(* Logix 5000 AddOnInstructionDefinition export Banner_TL70Pro_PD_v4; software revision 33.00 *)

TYPE Banner_TL70Pro_Adv_PD_Seg_v4 :   // Advanced process data set for a TL70 Pro Segment.
STRUCT
   Color_1 : SINT;   // 0 = Green, 1 = Red, 2 = Orange, 3 = Amber, 4 = Yellow, 5 = Lime Green, 6 = Spring Green, 7 = Cyan, 8 = Sky Blue, 9 = Blue, 10 = Violet, 11 = Magenta, 12 = Rose, 13 = White, 14 = Custom, 15 = Custom 2
   Color_1_Intensity : SINT;   // 0 = High, 1 = Low, 2 = Medium, 3 = Off, 4 = Custom
   Animation_Type : SINT;   // 0 = Off, 1 = Steady, 2 = Flash, 3 = Two Color, 4 = Half/Half, 5 = Half/Half Rotate, 6 = Chase, 7 = Intesnity Sweep
   Speed : SINT;   // 0 = Medium, 1 = Fast, 2 = Slow, 3 = Custom
   Pulse_Pattern : SINT;   // 0 = Normal, 1 = Strobe, 2 = Three Pulse, 3 = SOS, 4 = Random
   Color_2 : SINT;   // 0 = Green, 1 = Red, 2 = Orange, 3 = Amber, 4 = Yellow, 5 = Lime Green, 6 = Spring Green, 7 = Cyan, 8 = Sky Blue, 9 = Blue, 10 = Violet, 11 = Magenta, 12 = Rose, 13 = White, 14 = Custom, 15 = Custom 2
   Color_2_Instensity : SINT;   // 0 = High, 1 = Low, 2 = Medium, 3 = Off, 4 = Custom
END_STRUCT
END_TYPE

TYPE Banner_TL70Pro_Adv_PDIO_v4 :   // Advanced process data set for a TL70 Pro IO-Link unit.
STRUCT
   Segment_1 : Banner_TL70Pro_Adv_PD_Seg_v4;   // Advanced process data set for a TL70 Segment.
   Segment_2 : Banner_TL70Pro_Adv_PD_Seg_v4;   // Advanced process data set for a TL70 Segment.
   Segment_3 : Banner_TL70Pro_Adv_PD_Seg_v4;   // Advanced process data set for a TL70 Segment.
   Segment_4 : Banner_TL70Pro_Adv_PD_Seg_v4;   // Advanced process data set for a TL70 Segment.
   Segment_5 : Banner_TL70Pro_Adv_PD_Seg_v4;   // Advanced process data set for a TL70 Segment.
   Segment_6 : Banner_TL70Pro_Adv_PD_Seg_v4;   // Advanced process data set for a TL70 Segment.
   Audible : SINT;   // 0 = Off, 1 = On
END_STRUCT
END_TYPE

TYPE Banner_TL70Pro_Gauge_PD_v4 :   // Gauge mode process data set for a TL70 Pro IO-Link unit.
STRUCT
   Gauge_Value : INT;
   Audible : SINT;   // 0 = Off, 1 = On, 2 = Advanced
END_STRUCT
END_TYPE

TYPE Banner_TL70Pro_Level_PD_v4 :   // LeveL process data set for a TL70 Pro IO-Link unit.
STRUCT
   Level_Mode_Value : DINT;   // 0 to 65535. 0 = no lights on while 65535 = all lights on.
   Audible : SINT;   // 0 = Off, 1 = On
END_STRUCT
END_TYPE

TYPE Banner_TL70Pro_PDIO_v4 :   // Process data for a Banner TL70 Pro unit. This includes four process data types.
STRUCT
   Segment_PD : Banner_TL70Pro_Segment_PD_v4;
   Run_PD : Banner_TL70Pro_Run_PD_v4;
   Level_PD : Banner_TL70Pro_Level_PD_v4;
   Gauge_PD : Banner_TL70Pro_Gauge_PD_v4;
   Advanced_PD : Banner_TL70Pro_Adv_PDIO_v4;
   Transfer_Data : SINT[20];   // Data array to send the correct state of the process data output to the IO-Link master.
END_STRUCT
END_TYPE

TYPE Banner_TL70Pro_Run_PD_v4 :   // Run mode process data set for a TL70 Pro IO-Link unit.
STRUCT
   Animation : SINT;   // 0 = Off, 1 = Steady, 2 = Flash, 3 = Two Color, 4 = Half/Half, 5 = Half/Half Rotate, 6 = Chase, 7 = Intesnity Sweep, 8 = Scroll, 9 = Bounce, 10 = Demo
   Color_1 : SINT;   // 0 = Green, 1 = Red, 2 = Orange, 3 = Amber, 4 = Yellow, 5 = Lime Green, 6 = Spring Green, 7 = Cyan, 8 = Sky Blue, 9 = Blue, 10 = Violet, 11 = Magenta, 12 = Rose, 13 = White, 14 = Custom, 15 = Custom 2
   Color_1_Intensity : SINT;   // 0 = High, 1 = Low, 2 = Medium, 3 = Off, 4 = Custom
   Speed : SINT;   // 0 = Medium, 1 = Fast, 2 = Slow, 3 = Custom
   Pulse_Pattern : SINT;   // 0 = Normal, 1 = Strobe, 2 = Three Pulse, 3 = SOS, 4 = Random
   Color_2 : SINT;   // 0 = Green, 1 = Red, 2 = Orange, 3 = Amber, 4 = Yellow, 5 = Lime Green, 6 = Spring Green, 7 = Cyan, 8 = Sky Blue, 9 = Blue, 10 = Violet, 11 = Magenta, 12 = Rose, 13 = White, 14 = Custom, 15 = Custom 2
   Color_2_Intensity : SINT;   // 0 = High, 1 = Low, 2 = Medium, 3 = Off, 4 = Custom
   Scroll_Bounce_Style : SINT;   // 0 = Solid, 1 = Tail, 2 = Ripple
   Width_of_Color_1 : SINT;   // 1 to 100 percent
   Direction : SINT;   // 0 = Up, 1 = Down
   Audible : SINT;   // 0 = Off, 1 = On
END_STRUCT
END_TYPE

TYPE Banner_TL70Pro_Segment_PD_v4 :   // Basic process data set for a TL70 Pro IO-Link unit.
STRUCT
   Segment_1 : SINT;   // 0 = Off, 1 = On, 2 = Flash, 3 = Animation Type
   Segment_2 : SINT;   // 0 = Off, 1 = On, 2 = Flash, 3 = Animation Type
   Segment_3 : SINT;   // 0 = Off, 1 = On, 2 = Flash, 3 = Animation Type
   Segment_4 : SINT;   // 0 = Off, 1 = On, 2 = Flash, 3 = Animation Type
   Segment_5 : SINT;   // 0 = Off, 1 = On, 2 = Flash, 3 = Animation Type
   Segment_6 : SINT;   // 0 = Off, 1 = On, 2 = Flash, 3 = Animation Type
   Audible : SINT;   // 0 = Off, 1 = On
END_STRUCT
END_TYPE

ADD_ON_INSTRUCTION Banner_TL70Pro_Adv_PD_v4   (* revision 4.0, vendor Banner Engineering *)
// AOI converts the Advanced process and places it into the correct bytes for transfer to the IO-Link master.
VAR_IN_OUT
   Segment : Banner_TL70Pro_Adv_PD_Seg_v4; {required}
   Byte_1 : SINT; {required}
   Byte_2 : SINT; {required}
   Byte_3 : SINT; {required}
END_VAR

ROUTINE Logic   (* ladder *)
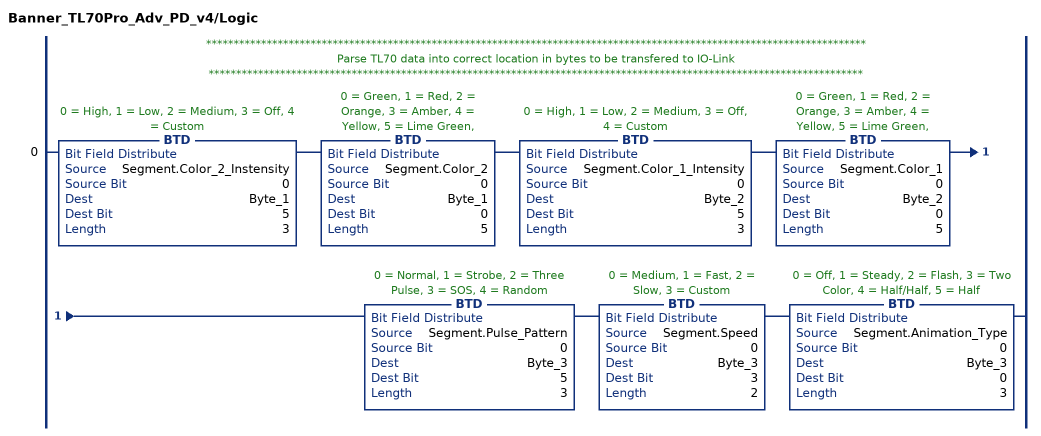
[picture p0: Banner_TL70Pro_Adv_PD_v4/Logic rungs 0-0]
   // ************************************************************************************************************************
   // Parse TL70 data into correct location in bytes to be transfered to IO-Link
   // ***********************************************************************************************************************
   0: BTD(Segment.Color_2_Instensity,0,Byte_1,5,3)BTD(Segment.Color_2,0,Byte_1,0,5)BTD(Segment.Color_1_Intensity,0,Byte_2,5,3)BTD(Segment.Color_1,0,Byte_2,0,5)BTD(Segment.Pulse_Pattern,0,Byte_3,5,3)BTD(Segment.Speed,0,Byte_3,3,2)BTD(Segment.Animation_Type,0,Byte_3,0,3);
END_ROUTINE
END_ADD_ON_INSTRUCTION

ADD_ON_INSTRUCTION Banner_TL70Pro_PD_v4   (* revision 4.0, vendor Banner Engineering *)
// Takes the raw SINT information and converts that data into actual information.
VAR_IN_OUT
   PDIO : Banner_TL70Pro_PDIO_v4; {required}
END_VAR
VAR_INPUT
   Byte_Swap : BOOL; {required}   // Swap the LSB and the MSB with each other.
   Operation_Mode : INT; {required}   // 0 = Segment, 1 = Run, 2 = Level, 3 = Gauge, 4 = Advanced
END_VAR
VAR
   Temp_Measurement : DINT; {access None}
   Data_Byte : SINT[20]; {access None}
   Temp_Data : SINT[20]; {access None}
   AOI_Status : Banner_TL70Pro_Adv_PD_v4[10]; {access None}
END_VAR

ROUTINE Logic   (* ladder *)
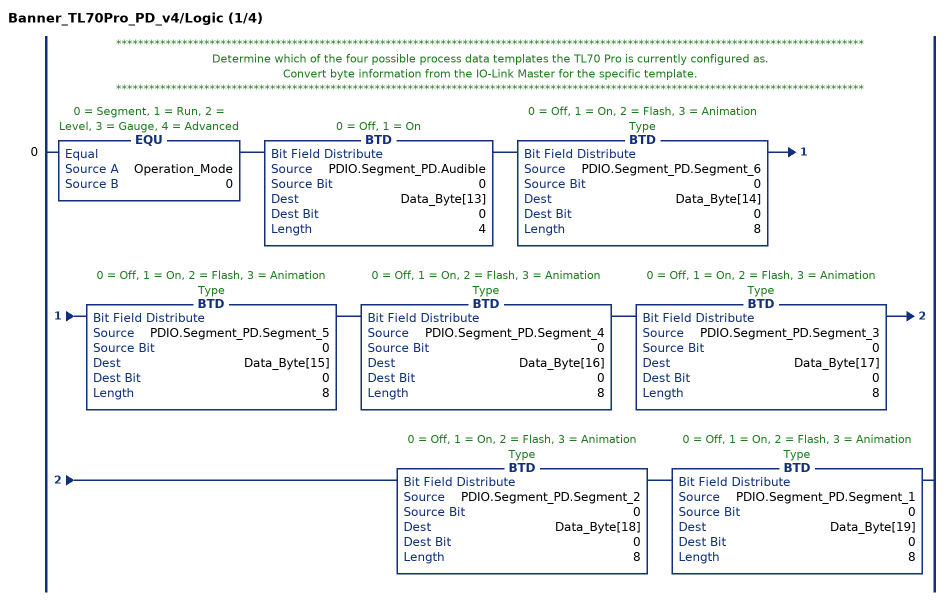
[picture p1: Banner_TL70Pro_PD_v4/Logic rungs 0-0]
   // ****************************************************************************************************************************************
   // Determine which of the four possible process data templates the TL70 Pro is currently configured as.
   // Convert byte information from the IO-Link Master for the specific template.
   // ****************************************************************************************************************************************
   0: EQU(Operation_Mode,0)BTD(PDIO.Segment_PD.Audible,0,Data_Byte[13],0,4)BTD(PDIO.Segment_PD.Segment_6,0,Data_Byte[14],0,8)BTD(PDIO.Segment_PD.Segment_5,0,Data_Byte[15],0,8)BTD(PDIO.Segment_PD.Segment_4,0,Data_Byte[16],0,8)BTD(PDIO.Segment_PD.Segment_3,0,Data_Byte[17],0,8)BTD(PDIO.Segment_PD.Segment_2,0,Data_Byte[18],0,8)BTD(PDIO.Segment_PD.Segment_1,0,Data_Byte[19],0,8);
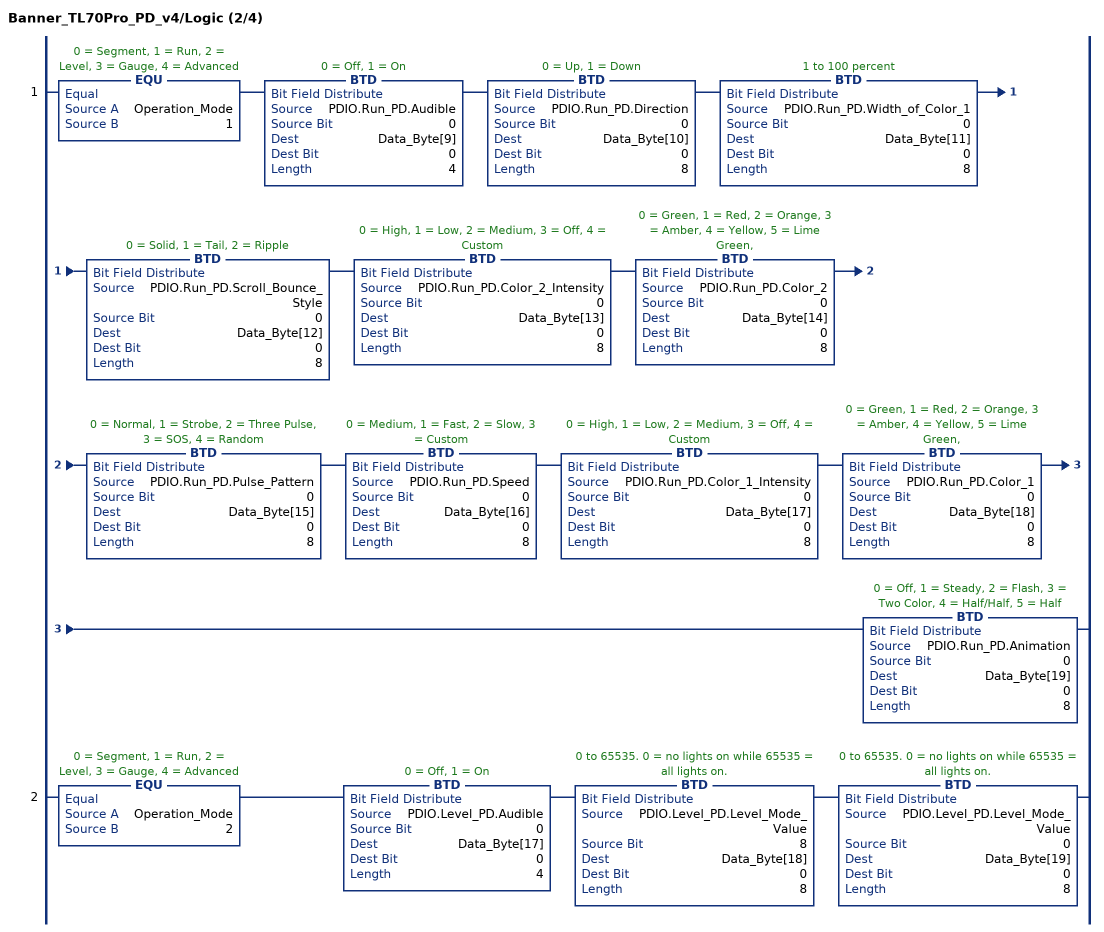
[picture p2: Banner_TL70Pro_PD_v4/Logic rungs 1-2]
   1: EQU(Operation_Mode,1)BTD(PDIO.Run_PD.Audible,0,Data_Byte[9],0,4)BTD(PDIO.Run_PD.Direction,0,Data_Byte[10],0,8)BTD(PDIO.Run_PD.Width_of_Color_1,0,Data_Byte[11],0,8)BTD(PDIO.Run_PD.Scroll_Bounce_Style,0,Data_Byte[12],0,8)BTD(PDIO.Run_PD.Color_2_Intensity,0,Data_Byte[13],0,8)BTD(PDIO.Run_PD.Color_2,0,Data_Byte[14],0,8)BTD(PDIO.Run_PD.Pulse_Pattern,0,Data_Byte[15],0,8)BTD(PDIO.Run_PD.Speed,0,Data_Byte[16],0,8)BTD(PDIO.Run_PD.Color_1_Intensity,0,Data_Byte[17],0,8)BTD(PDIO.Run_PD.Color_1,0,Data_Byte[18],0,8)BTD(PDIO.Run_PD.Animation,0,Data_Byte[19],0,8);
   2: EQU(Operation_Mode,2)BTD(PDIO.Level_PD.Audible,0,Data_Byte[17],0,4)BTD(PDIO.Level_PD.Level_Mode_Value,8,Data_Byte[18],0,8)BTD(PDIO.Level_PD.Level_Mode_Value,0,Data_Byte[19],0,8);
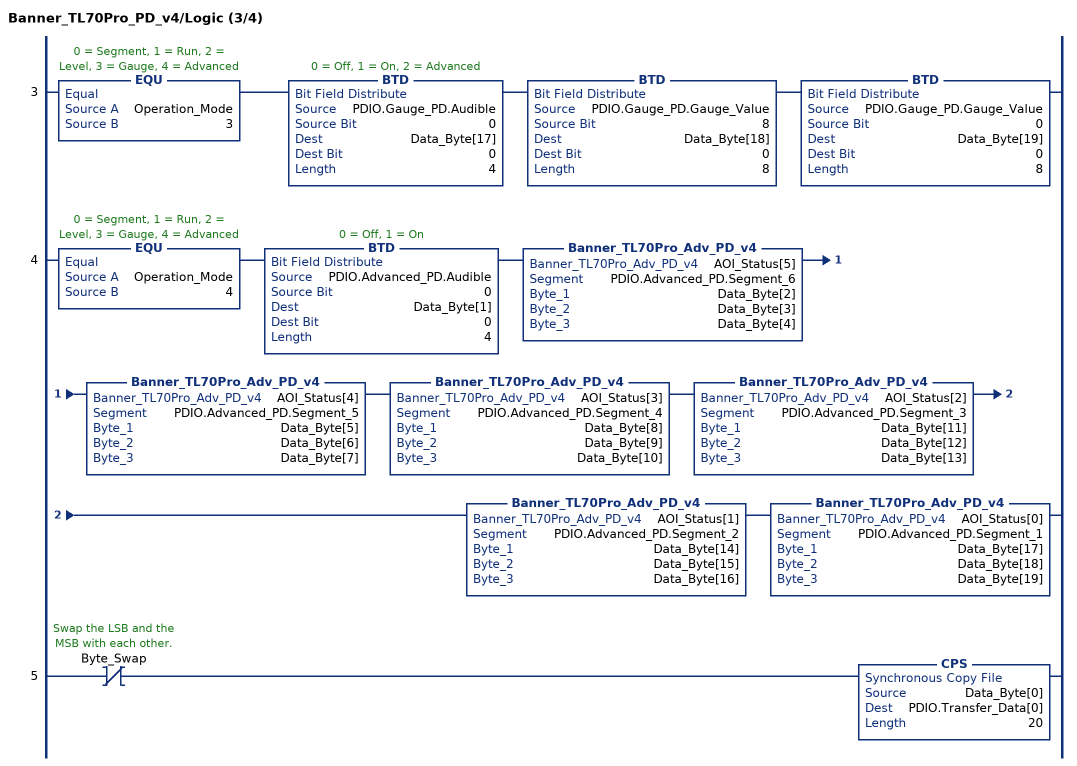
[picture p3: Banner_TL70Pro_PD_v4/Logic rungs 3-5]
   3: EQU(Operation_Mode,3)BTD(PDIO.Gauge_PD.Audible,0,Data_Byte[17],0,4)BTD(PDIO.Gauge_PD.Gauge_Value,8,Data_Byte[18],0,8)BTD(PDIO.Gauge_PD.Gauge_Value,0,Data_Byte[19],0,8);
   4: EQU(Operation_Mode,4)BTD(PDIO.Advanced_PD.Audible,0,Data_Byte[1],0,4)Banner_TL70Pro_Adv_PD_v4(AOI_Status[5],PDIO.Advanced_PD.Segment_6,Data_Byte[2],Data_Byte[3],Data_Byte[4])Banner_TL70Pro_Adv_PD_v4(AOI_Status[4],PDIO.Advanced_PD.Segment_5,Data_Byte[5],Data_Byte[6],Data_Byte[7])Banner_TL70Pro_Adv_PD_v4(AOI_Status[3],PDIO.Advanced_PD.Segment_4,Data_Byte[8],Data_Byte[9],Data_Byte[10])Banner_TL70Pro_Adv_PD_v4(AOI_Status[2],PDIO.Advanced_PD.Segment_3,Data_Byte[11],Data_Byte[12],Data_Byte[13])Banner_TL70Pro_Adv_PD_v4(AOI_Status[1],PDIO.Advanced_PD.Segment_2,Data_Byte[14],Data_Byte[15],Data_Byte[16])Banner_TL70Pro_Adv_PD_v4(AOI_Status[0],PDIO.Advanced_PD.Segment_1,Data_Byte[17],Data_Byte[18],Data_Byte[19]);
   5: XIO(Byte_Swap)CPS(Data_Byte[0],PDIO.Transfer_Data[0],20);
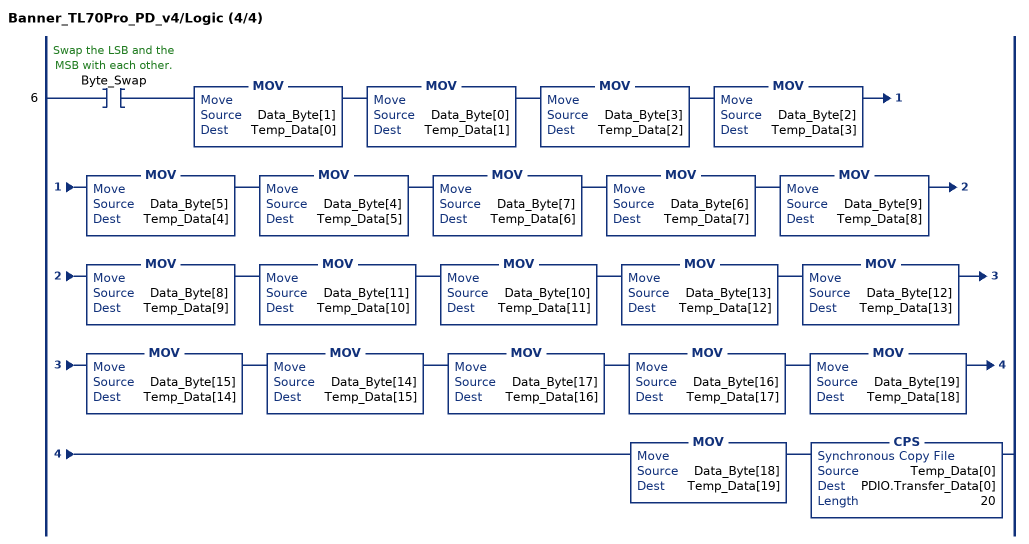
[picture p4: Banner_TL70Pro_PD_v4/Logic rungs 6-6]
   6: XIC(Byte_Swap)MOV(Data_Byte[1],Temp_Data[0])MOV(Data_Byte[0],Temp_Data[1])MOV(Data_Byte[3],Temp_Data[2])MOV(Data_Byte[2],Temp_Data[3])MOV(Data_Byte[5],Temp_Data[4])MOV(Data_Byte[4],Temp_Data[5])MOV(Data_Byte[7],Temp_Data[6])MOV(Data_Byte[6],Temp_Data[7])MOV(Data_Byte[9],Temp_Data[8])MOV(Data_Byte[8],Temp_Data[9])MOV(Data_Byte[11],Temp_Data[10])MOV(Data_Byte[10],Temp_Data[11])MOV(Data_Byte[13],Temp_Data[12])MOV(Data_Byte[12],Temp_Data[13])MOV(Data_Byte[15],Temp_Data[14])MOV(Data_Byte[14],Temp_Data[15])MOV(Data_Byte[17],Temp_Data[16])MOV(Data_Byte[16],Temp_Data[17])MOV(Data_Byte[19],Temp_Data[18])MOV(Data_Byte[18],Temp_Data[19])CPS(Temp_Data[0],PDIO.Transfer_Data[0],20);
END_ROUTINE
END_ADD_ON_INSTRUCTION
